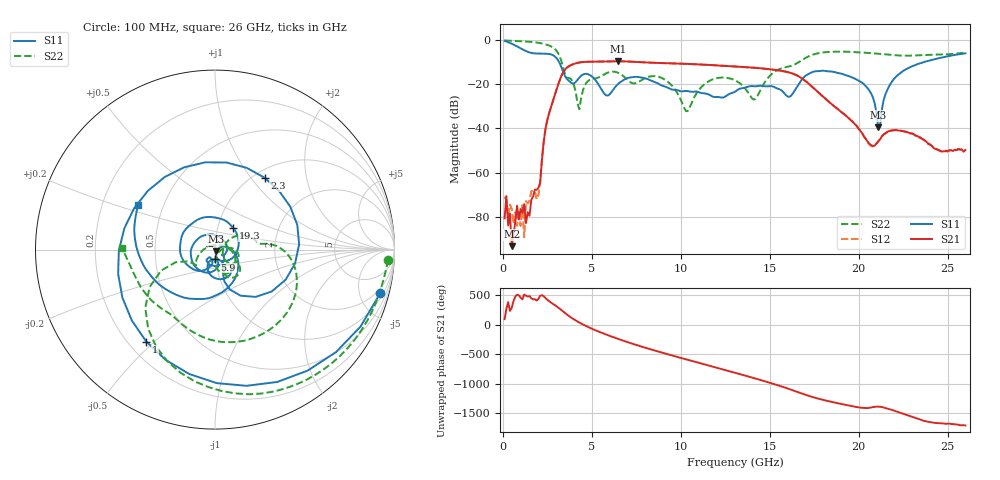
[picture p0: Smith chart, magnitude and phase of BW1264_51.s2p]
!Keysight Technologies,N5245B,MY57181159,A.13.60.06
!Date: Friday, December 18, 2020 23:54:46
!Correction: S11(Full 2 Port(1,2))
!S21(Full 2 Port(1,2))
!S12(Full 2 Port(1,2))
!S22(Full 2 Port(1,2))
!S2P File: Measurements: S11, S21, S12, S22:
# Hz S  dB  R 50
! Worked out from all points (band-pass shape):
!   260 points, 100 MHz to 26 GHz, reference 50 ohm
!   highest |S21| = -9.71 dB at 6.5 GHz (marker M1); lowest = -93.2 dB at 500 MHz (marker M2)
!   |S21| within 3 dB of the highest: 3.584 GHz to 14.26 GHz (10.68 GHz wide, 120 % of centre)
!   lowest |S11| = -39.5 dB at 21.1 GHz (marker M3), VSWR 1.02, Z = 50.4 - j0.983 ohm
!   |S11| at or under -10 dB: 3.156 GHz to 23.69 GHz (20.54 GHz wide, 153 % of centre)
!   |S22| runs from -32.3 to -0.3 dB; largest |S21 - S12| = 0.00061
!   S11 on the Smith chart (normalised r, x): 100 MHz: 1.43, -7.44; 1 GHz: 0.27, -0.47; 2.3 GHz: 1.12, +1.17; 5.9 GHz: 0.99, -0.11; 19.3 GHz: 1.19, +0.29; 26 GHz: 0.36, +0.23
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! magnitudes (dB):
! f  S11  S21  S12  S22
! 100 MHz  -0.4  -80.7  -70.9  -0.3
! 200 MHz  -0.7  -70.6  -72.4  -0.4
! 500 MHz  -1.8  -93.2  -76.4  -0.5
! 1 GHz  -3.9  -76.5  -84.0  -0.6
! 2 GHz  -6.2  -66.9  -70.2  -1.4
! 2.3 GHz  -6.3  -46.0  -45.7  -1.8
! 3.3 GHz  -12.6  -16.2  -16.2  -9.8
! 4.3 GHz  -17.1  -10.3  -10.3  -31.4
! 4.5 GHz  -15.7  -10.1  -10.1  -22.9
! 5.9 GHz  -25.2  -9.8  -9.8  -14.9
! 6.5 GHz  -19.8  -9.7  -9.7  -15.0
! 8.8 GHz  -20.1  -10.5  -10.5  -16.8
! 10.3 GHz  -23.1  -10.9  -10.9  -32.3
! 13.1 GHz  -23.2  -12.1  -12.1  -18.5
! 14.1 GHz  -21.0  -12.6  -12.6  -27.0
! 16.1 GHz  -25.8  -14.8  -14.8  -12.0
! 17.4 GHz  -14.6  -21.3  -21.3  -6.8
! 19.3 GHz  -16.1  -34.4  -34.4  -5.4
! 20.6 GHz  -22.9  -47.0  -47.3  -6.0
! 21.1 GHz  -39.5  -46.0  -45.9  -6.3
! 21.7 GHz  -21.2  -41.3  -41.2  -6.8
! 26 GHz  -6.1  -49.8  -50.0  -5.7
